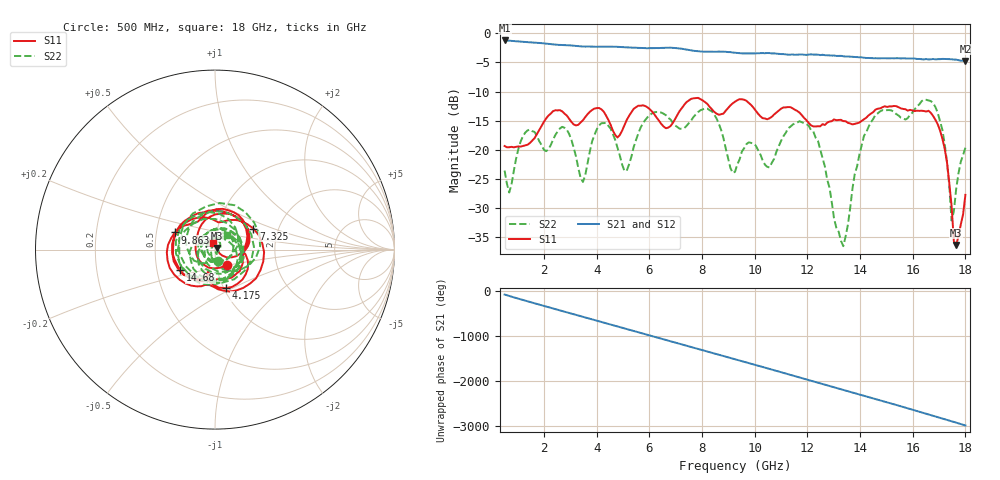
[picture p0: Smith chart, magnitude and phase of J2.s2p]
!Agilent Technologies,N5230A,MY45001360,A.07.50.67
!Agilent N5230A: A.07.50.67
!Date: Tuesday, April 16, 2024 15:48:43
!Correction: S11(Full 2 Port(1,2))
!S21(Full 2 Port(1,2))
!S12(Full 2 Port(1,2))
!S22(Full 2 Port(1,2))
!S2P File: Measurements: S11, S21, S12, S22:
# Hz S  dB  R 50
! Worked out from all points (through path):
!   201 points, 500 MHz to 18 GHz, reference 50 ohm
!   highest |S21| = -1.24 dB at 500 MHz (marker M1); lowest = -4.8 dB at 18 GHz (marker M2)
!   group delay of S21, straight-line fit = 458 ps
!   lowest |S11| = -36.3 dB at 17.65 GHz (marker M3), VSWR 1.03, Z = 51.2 + j0.965 ohm
!   |S11| at or under -10 dB: start of sweep to end of sweep
!   |S22| runs from -36.5 to -11.4 dB; largest |S21 - S12| = 0.0077
!   S11 on the Smith chart (normalised r, x): 500 MHz: 1.13, -0.19; 4.175 GHz: 1.02, -0.46; 7.325 GHz: 1.49, +0.37; 9.863 GHz: 0.63, +0.13; 14.68 GHz: 0.66, -0.16; 18 GHz: 0.97, +0.08
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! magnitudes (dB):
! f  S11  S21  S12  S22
! 500 MHz  -19.3  -1.2  -1.2  -23.5
! 675 MHz  -19.5  -1.3  -1.3  -27.3
! 1.288 GHz  -19.2  -1.5  -1.5  -17.0
! 2.688 GHz  -13.4  -2.0  -2.0  -16.0
! 3.475 GHz  -14.9  -2.3  -2.3  -25.5
! 4.175 GHz  -13.0  -2.3  -2.3  -15.4
! 5.138 GHz  -14.9  -2.4  -2.4  -23.6
! 6.362 GHz  -15.0  -2.6  -2.5  -13.5
! 7.325 GHz  -12.2  -2.7  -2.7  -16.3
! 8.375 GHz  -13.1  -3.2  -3.2  -13.4
! 9.25 GHz  -11.7  -3.4  -3.3  -23.8
! 9.863 GHz  -12.3  -3.5  -3.5  -18.8
! 10.56 GHz  -14.6  -3.4  -3.4  -23.0
! 12.22 GHz  -16.0  -3.7  -3.6  -16.8
! 13.36 GHz  -15.1  -4.0  -3.9  -36.5
! 14.15 GHz  -14.8  -4.2  -4.2  -17.6
! 14.68 GHz  -12.9  -4.3  -4.3  -13.7
! 15.11 GHz  -12.5  -4.3  -4.3  -13.2
! 16.95 GHz  -15.6  -4.4  -4.4  -13.6
! 17.48 GHz  -29.5  -4.5  -4.4  -32.1
! 17.65 GHz  -36.3  -4.5  -4.6  -26.7
! 18 GHz  -27.7  -4.8  -4.8  -19.6
